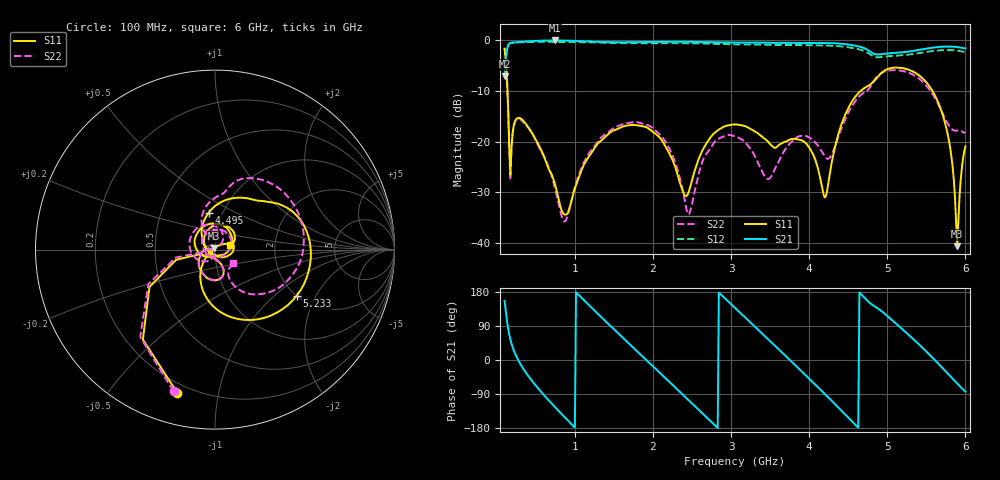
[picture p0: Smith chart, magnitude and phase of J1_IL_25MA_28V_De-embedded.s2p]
!Keysight Technologies,N5242B,MY61256241,Z.15.82.127
!Date: Friday, August 25, 2023 02:26:26
!Correction: S11(C  4-Port  )
!S21(C  4-Port  )
!S12(C  4-Port  )
!S22(C  4-Port  )
!S2P File: Measurements: S11, S21, S12, S22:
# Hz S  dB  R 50
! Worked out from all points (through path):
!   401 points, 100 MHz to 6 GHz, reference 50 ohm
!   highest |S21| = -0.07 dB at 749 MHz (marker M1); lowest = -7.1 dB at 100 MHz (marker M2)
!   group delay of S21, straight-line fit = 555 ps
!   lowest |S11| = -40.6 dB at 5.897 GHz (marker M3), VSWR 1.02, Z = 49.6 + j0.826 ohm
!   |S11| at or under -10 dB: 136.2 MHz to 4.66 GHz (4.524 GHz wide, 189 % of centre); 5.578 GHz to end of sweep
!   |S22| runs from -35.7 to -1.7 dB; largest |S21 - S12| = 0.067
!   S11 on the Smith chart (normalised r, x): 100 MHz: 0.15, -0.76; 4.495 GHz: 0.86, +0.37; 5.233 GHz: 2.00, -1.42; 6 GHz: 1.19, +0.06
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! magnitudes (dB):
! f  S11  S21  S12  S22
! 100 MHz  -1.7  -7.1  -7.1  -1.7
! 188.5 MHz  -21.1  -0.5  -0.5  -21.4
! 321.2 MHz  -15.6  -0.3  -0.4  -15.8
! 749 MHz  -28.6  -0.1  -0.3  -29.4
! 881.8 MHz  -34.4  -0.1  -0.4  -35.6
! 1.088 GHz  -25.5  -0.2  -0.4  -25.1
! 1.59 GHz  -17.2  -0.4  -0.6  -16.7
! 2.076 GHz  -19.0  -0.3  -0.6  -18.4
! 2.46 GHz  -29.8  -0.3  -0.6  -34.3
! 2.667 GHz  -20.8  -0.4  -0.7  -22.8
! 3.05 GHz  -16.6  -0.5  -0.9  -19.0
! 3.478 GHz  -20.1  -0.5  -0.9  -27.4
! 3.802 GHz  -19.4  -0.6  -1.0  -19.6
! 4.038 GHz  -22.2  -0.6  -1.0  -19.6
! 4.215 GHz  -30.6  -0.6  -1.1  -23.2
! 4.495 GHz  -13.6  -0.9  -1.4  -14.4
! 5.027 GHz  -5.6  -2.6  -3.2  -6.0
! 5.233 GHz  -5.6  -2.3  -2.9  -6.2
! 5.69 GHz  -13.8  -1.3  -2.0  -13.8
! 5.808 GHz  -21.5  -1.3  -2.0  -17.2
! 5.897 GHz  -40.6  -1.4  -2.1  -17.8
! 6 GHz  -20.9  -1.6  -2.3  -18.1
